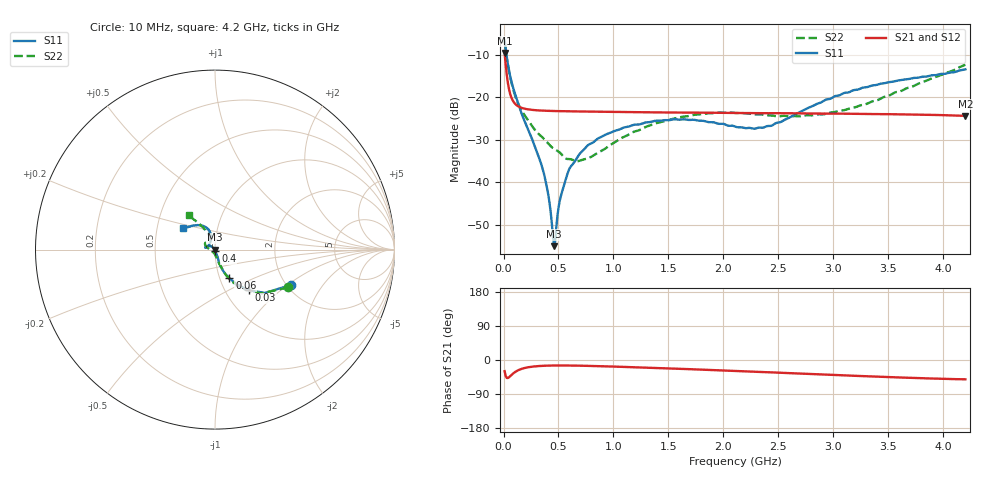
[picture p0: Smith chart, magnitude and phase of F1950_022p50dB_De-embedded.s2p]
! Integrated Device Technology
! Corporate Headquarters
! 6024 Silver Creek Valley Road
! San Jose, CA 95138  USA
! Phone:  1-408-284-8200
! Toll Free:  1-800-223-1366
! Webpage:  http://www.idt.com/
! Timing and RF Division
! 515 Groton Road, Suite 102
! Westford, MA 01886-6024
! Device:  F1950
! Description: 7-bit 0.25 dB Digital Step Attenuator
! Frequency:  150.0 -  4000.00 MHz
! Package:  4x4 mm Thin QFN Plastic Package: 24 pin
! Ports:  2 RF, 12 DC
!  Pin  1  = D0
!  Pin  2  = VDD
!  Pin  3  = Vmode
!  Pin  4  = GND
!  Pin  5  = RF1  =  Port 1
!  Pin  6  = GND
!  Pin  7  = GND
!  Pin  8  = GND
!  Pin  9  = GND
!  Pin 10  = GND
!  Pin 11  = GND
!  Pin 12  = GND
!  Pin 13  = GND
!  Pin 14  = RF2  =  Port 2
!  Pin 15  = GND
!  Pin 16  = LE
!  Pin 17  = CLK
!  Pin 18  = DATE
!  Pin 19  = D6
!  Pin 20  = D5
!  Pin 21  = D4
!  Pin 22  = D3
!  Pin 23  = D2
!  Pin 24  = D1
! State:  90
! Atten State:  22.50 dB
! Voltage:  +5.00 Volts
! Current:  Not Measured mA
! Data:  The device was measured on a the F195X evaluation board which has
!  individual transmission lines to the RF pins.  Data was collected
!  using a calibrated network analyzer.  The evaluation board was
!  de-embedded using a TRL calibration technique.
!  The reference plane is the edge of the package pin.
! Misc:  Board 2019
!  Action Tracker AT0250
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# GHz S dB R 50
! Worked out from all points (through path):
!   420 points, 10 MHz to 4.2 GHz, reference 50 ohm
!   highest |S21| = -9.59 dB at 10 MHz (marker M1); lowest = -24.4 dB at 4.2 GHz (marker M2)
!   group delay of S21, straight-line fit = 24.2 ps
!   lowest |S11| = -55.1 dB at 460 MHz (marker M3), VSWR 1.00, Z = 49.9 - j0.0957 ohm
!   |S11| at or under -10 dB: 27.04 MHz to end of sweep
!   |S22| runs from -35.1 to -6.8 dB; largest |S21 - S12| = 0.00012
!   S11 on the Smith chart (normalised r, x): 10 MHz: 2.09, -1.06; 30 MHz: 1.29, -0.64; 60 MHz: 1.11, -0.36; 400 MHz: 1.00, -0.02; 4.2 GHz: 0.68, +0.17
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0.01  -6.65 -25.2  -9.59 -29.4  -9.59 -29.4  -6.76 -27.3
0.03  -10.56 -49.9  -14.79 -47.3  -14.79 -47.3  -10.89 -52.2
0.06  -14.99 -63.3  -19.19 -42.9  -19.19 -42.9  -15.18 -64.8
0.1  -18.87 -70.2  -21.40 -32.8  -21.40 -32.8  -19.23 -70.1
0.16  -23.54 -72.2  -22.47 -23.9  -22.47 -23.9  -22.91 -75.1
0.33  -34.78 -71.6  -23.14 -15.8  -23.14 -15.8  -28.92 -83.9
0.4  -41.95 -74.9  -23.22 -14.9  -23.22 -14.9  -30.72 -87.1
0.45  -52.91 -112.6  -23.26 -14.6  -23.26 -14.6  -32.02 -93.5
0.46  -55.08 -147.0  -23.27 -14.5  -23.26 -14.5  -32.21 -95.2
0.48  -50.61 157.2  -23.28 -14.5  -23.27 -14.5  -32.50 -98.2
0.52  -43.45 141.8  -23.30 -14.4  -23.30 -14.4  -33.27 -101.8
0.58  -38.15 136.2  -23.33 -14.5  -23.33 -14.5  -34.57 -114.3
0.71  -32.88 138.5  -23.38 -15.1  -23.38 -15.1  -34.78 -139.6
1  -28.06 148.4  -23.48 -17.3  -23.48 -17.3  -30.81 179.9
1.41  -25.56 163.4  -23.59 -21.3  -23.59 -21.3  -25.97 161.5
1.73  -25.33 168.8  -23.65 -24.6  -23.65 -24.6  -24.17 153.2
2.11  -26.97 158.7  -23.73 -29.1  -23.72 -29.1  -23.74 143.5
2.43  -26.77 127.3  -23.77 -32.5  -23.77 -32.6  -24.29 133.0
2.81  -22.12 106.0  -23.84 -37.1  -23.83 -37.2  -24.28 117.8
3.1  -19.00 107.5  -23.90 -40.6  -23.89 -40.6  -23.05 112.7
3.51  -16.45 117.8  -24.01 -45.1  -24.00 -45.2  -19.60 114.1
4.2  -13.45 145.9  -24.40 -51.0  -24.40 -51.0  -12.37 127.3
